FUNCTION_BLOCK FB_Module
// Base class of modules with axis and buttons for manual control
VAR_INPUT
		(***** Enables *****)
	bComprAirEnabled			: BOOL;						// Enable of compressed air
	bAxisEnable					: BOOL;						// Enable of axis
	bSensorEnable				: BOOL;						// Enable of sensor
	bManualAxisEnable			: BOOL;						// Enable of manual axis control
		(***** State variables *****)
	bStarting					: BOOL;						// True if machine is in state STARTING
	bHalt						: BOOL;						// True if machine is in state ABORTING or STOPPING
	bReset						: BOOL;						// True if machine is in state RESETTING
		(**** Variables of axis *****)
	lrAxisVelo					: LREAL;					// Velocity of axis
	bButtonAxisFwIn				: BOOL;
	bButtonAxisBwIn				: BOOL;	
END_VAR
VAR_OUTPUT
	bAxisMoves					: BOOL;						// True if axis is moving
	bButtonAxisFwOut			: BOOL;
	bButtonAxisBwOut			: BOOL;				
	bStartingDone				: BOOL;						// True if module is started
	bHaltDone					: BOOL;						// True if module is stopped
	bResetDone					: BOOL;						// True if module is reset
	
		(***** Function block instance of FB_Axis *)
	fbAxis						: FB_Axis;
END_VAR
VAR
		(***** Manual axis control *****)
	fbButtonAxisFw				: FB_SignalHandlingIntern;	// To move axis forwards	
	fbButtonAxisBw				: FB_SignalHandlingIntern;	// To move axis backwards
	
(* ========================== COMMON VARIABLES =============================== *)	
	fbTriggerStartingStart		: R_TRIG;					// To diagnose rising edge of starting action starting
	fbTriggerHaltStart			: R_TRIG;					// To diagnose rising edge of starting halt
	fbTriggerResetStart			: R_TRIG;					// To diagnose rising edge of starting reset			
	bManualCylinderEnable		: BOOL;						// Enable of manual cylinder control	
	bMoved						: BOOL;
END_VAR

// =========================================================
;
// =========================================================

METHOD PUBLIC M_Enable
VAR_INPUT
END_VAR
// =========================================================
		// Axis control
		
fbAxis.bEnable := bAxisEnable;		// Setting variable to enable axis

fbAxis.M_Enable();					// Enabling axis

// =========================================================
		// Cylinder control
		
bManualCylinderEnable := bManualAxisEnable AND bComprAirEnabled;

// =========================================================
		// Axis control
		
fbButtonAxisFw.bEnable := bManualAxisEnable AND NOT fbButtonAxisBw.bOut;
fbButtonAxisBw.bEnable := bManualAxisEnable AND NOT fbButtonAxisFw.bOut;

// =========================================================
END_METHOD

METHOD PUBLIC M_Reset
VAR_INPUT
END_VAR
// =========================================================
		// Resetting variables

bMoved 		:= FALSE;
bHaltDone 	:= FALSE;
bHalt 		:= FALSE;

// =========================================================
		// Resetting axis

fbAxis.bDriveReset := fbTriggerResetStart.Q;		
						
fbAxis.M_Reset();

bResetDone := fbAxis.bResetDone;

// =========================================================
END_METHOD

METHOD PUBLIC M_Halt
VAR_INPUT
END_VAR
// =========================================================
		// Halting axis

fbAxis.bHalt := bHalt;				// Setting variable to halt axis

fbAxis.M_Halt();					// Halting axis

IF bHalt THEN
	bHaltDone := fbAxis.bHaltDone;	// Getting halt state
ELSE
	bHaltDone := FALSE;
END_IF

// =========================================================
END_METHOD

METHOD PUBLIC M_Stop
VAR_INPUT
END_VAR
// =========================================================
		// Stopping axis

fbAxis.bHalt := bHalt;						// Setting variable to halt axis

fbAxis.M_Stop();							// Stopping axis

IF bHalt THEN
	bHaltDone := fbAxis.bHaltDone;			// Getting halt state
ELSE
	bHaltDone := FALSE;
END_IF

// =========================================================
END_METHOD

METHOD PUBLIC M_Starting
VAR_INPUT
END_VAR
// =========================================================

fbTriggerStartingStart( CLK := bStarting );

IF fbTriggerStartingStart.Q THEN
	bStartingDone 		:= FALSE;
	fbAxis.lrVelocity 	:= lrAxisVelo;		// Setting velocity of axis
	M_ResetState();							// Resetting state variable
END_IF

IF fbAxis.bStatus THEN
	bStartingDone := TRUE;
END_IF

// =========================================================
END_METHOD

METHOD PROTECTED M_ResetState
VAR_INPUT
END_VAR
// =========================================================

;

// =========================================================
END_METHOD

METHOD PUBLIC M_Manual
VAR_INPUT
END_VAR
// =========================================================
	// Manual axis control
	
IF fbButtonAxisBw.bOut THEN				(* Button to move axis backwards pressed *)
	
	IF bHaltDone THEN
		bHaltDone := FALSE;							// Resetting bHaltDone
	END_IF
	
	IF NOT bMoved THEN
		bMoved := TRUE;
	END_IF
	
	fbAxis.M_MoveBw();								// Move axis forwards
	
ELSIF fbButtonAxisFw.bOut THEN			(* Button to move axis forwards pressed *)
	
	IF bHaltDone THEN
		bHaltDone := FALSE;							// Resetting bHaltDone
	END_IF
	
	IF NOT bMoved THEN
		bMoved := TRUE;
	END_IF
	
	fbAxis.M_MoveFw();								// Move axis backwards
	
ELSIF NOT bHaltDone THEN				(* No button is pressed and halt is not done *)
	
	IF bMoved THEN								(* Request halt if axis has moved *)
		
		IF NOT bHalt THEN
			bHalt := TRUE;							// Setting variable to halt axis
		END_IF
		
		M_Halt();
	END_IF
	
ELSIF bHalt THEN						(* Halt is done but still requested *)
	bHalt := FALSE;									// Resetting variable to halt axis
	
	M_Halt();
	
	bMoved := FALSE;
END_IF

// =========================================================
END_METHOD

METHOD PUBLIC M_SetOutput
VAR_INPUT
END_VAR
// =========================================================
		// Axis buttons and output variable for axis
		
fbButtonAxisFw.M_SetOutput();	
fbButtonAxisBw.M_SetOutput();

bAxisMoves := fbAxis.bMoves;				// Getting moving state

fbButtonAxisFw.bInput 	:= bButtonAxisFwIn;
fbButtonAxisBw.bInput	:= bButtonAxisBwIn;
bButtonAxisFwOut 		:= fbButtonAxisFw.bOut;
bButtonAxisBwOut		:= fbButtonAxisBw.bOut;

// =========================================================
END_METHOD

END_FUNCTION_BLOCK
